(* Logix 5000 AddOnInstructionDefinition export; software revision 16.04 *)

TYPE AKD_Status :   // All connections to the drive ethernet module are established and data is successfully transferring.
STRUCT
   Profile_In_Progress : BOOL;   // Profile Move In Progress
   Block_In_Execution : BOOL;   // Block In Execution
   On_Target_Position : BOOL;   // On Target Position (1=Current Position Equals Last Target Position)
   General_Fault : BOOL;   // General Fault
   Current_Direction : BOOL;   // Current Motor Direction (0=Reverse, 1=Forward)
   Home_Level : BOOL;   // Level of Home Input
   Reg_Level : BOOL;   // Level of Registration Input
   Enable : BOOL;   // State of Enable Output
   Fault_Input_Fault : BOOL;   // Fault Input Active
   Fwd_Limit : BOOL;   // Forward Input Active
   Rev_Limit : BOOL;   // Reverse Input Active
   Positive_Limit : BOOL;   // Positive Software Limit Exceeded
   Negative_Limit : BOOL;   // Negative Software Limit Exceeded
   FE_Fault : BOOL;   // Following Error Fault
   Block_Fault : BOOL;   // Block Execution Fault
   Load_Complete : BOOL;   // Command Message Successfully Loaded
END_STRUCT
END_TYPE

TYPE AKD_Axis :   // Axis Data:
STRUCT
   Control : AKD_Control;   // Control bits to send to the drive
   Status : AKD_Status;   // Status bits received from the drive
   Input : AB:ETHERNET_MODULE_SINT_64Bytes:I:0;   // Data from the drive
   Output : AB:ETHERNET_MODULE_SINT_64Bytes:O:0;   // Data to the drive
   ResponseMsgType : SINT;   // Response type contained in latest IO response from drive. Used to check for errors
   CommandTimeout : INT;   // Time to allow for command response from drive. Dependent on scan rate and communicaiton rate
   PositionFeedback : DINT;   // Actual Position Value
   VelocityFeedback : DINT;   // Actual Velocity Value
END_STRUCT
END_TYPE

TYPE AKD_Control :   // Send Explicit Message
STRUCT
   Load_Data_Start_Profile : BOOL;   // Load Command Data / Start Profile Move
   Start_Block : BOOL;   // Execute Command block or block chain
   Incremental : BOOL;   // Incremental Position (0=Absolute, 1=Incremental)
   Direction : BOOL;   // Direction in Velocity Mode (0=Reverse, 1=Forward)
   Smooth_Stop : BOOL;   // Smooth / Controlled Stop w/ Deceleration
   Hard_Stop : BOOL;   // Hard / Immediate Stop
   Reg_Arm : BOOL;   // Arm the Registration Input
   Enable : BOOL;   // Enable Output
END_STRUCT
END_TYPE

ADD_ON_INSTRUCTION AKD_Disable   (* revision 2.1, ExecutePrescan, ExecuteEnableInFalse *)
// Disable Drive
// Revision note:
// Don't error if Command_Timeout preset is 0
VAR_OUTPUT
   DN : BOOL; {visible}   // Command Successful
   ER : BOOL; {visible}   // Error
END_VAR
VAR_IN_OUT
   Axis : AKD_Axis; {required}
END_VAR
VAR
   Command_Timeout : TIMER;   // Timeout Timer
END_VAR

ROUTINE EnableInFalse   (* ladder *)
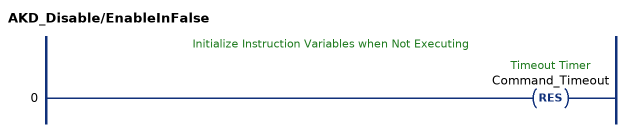
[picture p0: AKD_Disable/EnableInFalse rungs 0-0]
   // Initialize Instruction Variables when Not Executing
   0: RES(Command_Timeout);
END_ROUTINE

ROUTINE Logic   (* ladder *)
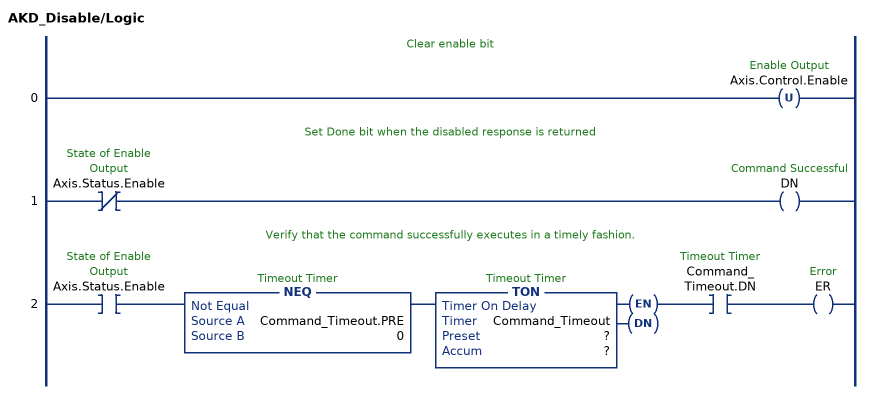
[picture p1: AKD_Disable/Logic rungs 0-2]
   // Clear enable bit
   0: OTU(Axis.Control.Enable);
   // Set Done bit when the disabled response is returned
   1: XIO(Axis.Status.Enable)OTE(DN);
   // Verify that the command successfully executes in a timely fashion.
   2: XIC(Axis.Status.Enable)NEQ(Command_Timeout.PRE,0)TON(Command_Timeout,?,?)XIC(Command_Timeout.DN)OTE(ER);
END_ROUTINE

ROUTINE Prescan   (* ladder *)
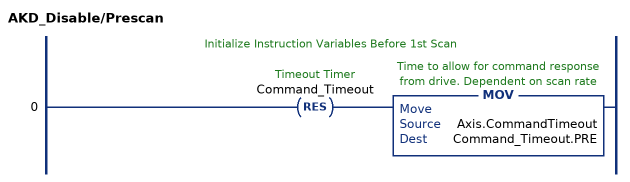
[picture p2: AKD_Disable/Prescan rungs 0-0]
   // Initialize Instruction Variables Before 1st Scan
   0: RES(Command_Timeout)MOV(Axis.CommandTimeout,Command_Timeout.PRE);
END_ROUTINE
END_ADD_ON_INSTRUCTION

ADD_ON_INSTRUCTION AKD_Set_Parameter   (* revision 2.0, ExecutePrescan, ExecuteEnableInFalse *)
// Set Drive Parameter
VAR_OUTPUT
   DN : BOOL; {visible}   // Command Successful
   ER : BOOL; {visible}   // Error
END_VAR
VAR_IN_OUT
   Axis : AKD_Axis; {required}
END_VAR
VAR_INPUT
   Parameter_Number : INT; {visible}   // See help (F1) for parameter list.
   Parameter_Value : DINT; {required}   // Parameter Value
END_VAR
VAR
   Command_Timeout : TIMER;   // Timeout Timer
   Command_Message_Type : SINT;   // Command Message Type
   Command_Axis_Number : SINT;   // Command Axis Number
   Step : SINT;
   Command_Bytes : SINT[8];
   OS_LoadStart : BOOL;
   Temp_Bytes : SINT[2];   // Temporary Bytes to Split into Command Bytes
END_VAR

ROUTINE EnableInFalse   (* ladder *)
// EnableIn_False
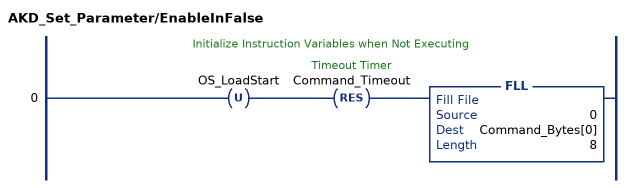
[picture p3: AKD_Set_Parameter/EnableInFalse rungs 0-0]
   // Initialize Instruction Variables when Not Executing
   0: OTU(OS_LoadStart)RES(Command_Timeout)FLL(0,Command_Bytes[0],8);
END_ROUTINE

ROUTINE Logic   (* ladder *)
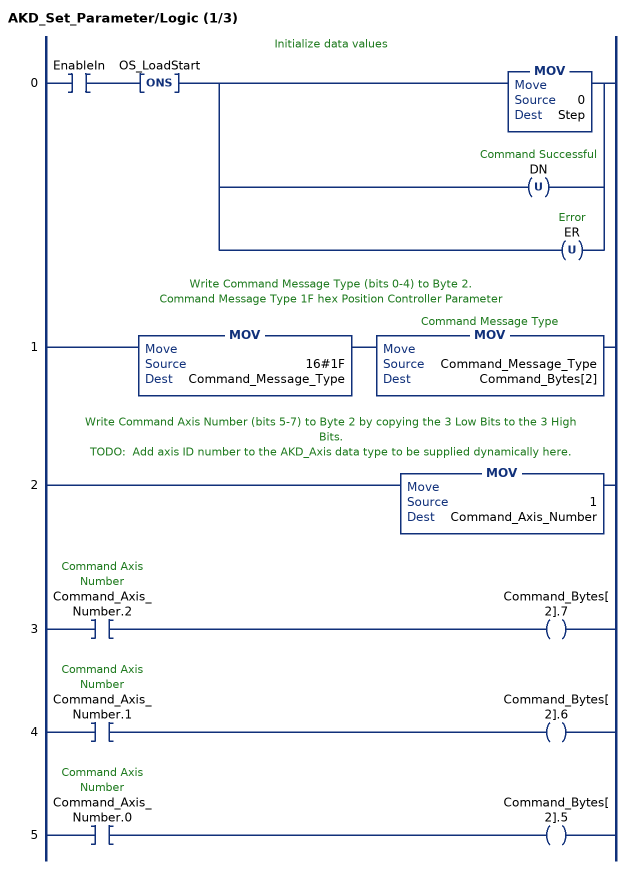
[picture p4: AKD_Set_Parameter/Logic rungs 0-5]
   // Initialize data values
   0: XIC(EnableIn)ONS(OS_LoadStart)[MOV(0,Step) ,OTU(DN) ,OTU(ER) ];
   // Write Command Message Type (bits 0-4) to Byte 2.
   // Command Message Type 1F hex Position Controller Parameter
   1: MOV(16#1F,Command_Message_Type)MOV(Command_Message_Type,Command_Bytes[2]);
   // Write Command Axis Number (bits 5-7) to Byte 2 by copying the 3 Low Bits to the 3 High Bits.
   // TODO:  Add axis ID number to the AKD_Axis data type to be supplied dynamically here.
   2: MOV(1,Command_Axis_Number);
   3: XIC(Command_Axis_Number.2)OTE(Command_Bytes[2].7);
   4: XIC(Command_Axis_Number.1)OTE(Command_Bytes[2].6);
   5: XIC(Command_Axis_Number.0)OTE(Command_Bytes[2].5);
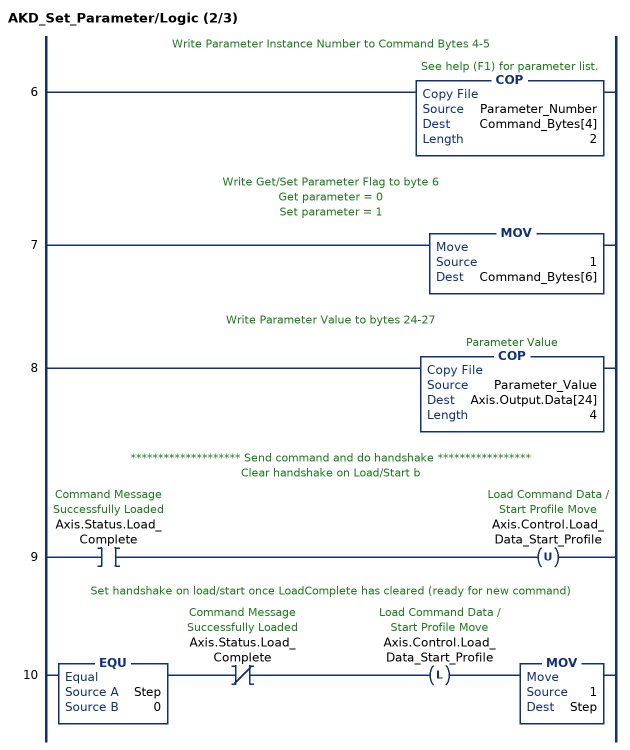
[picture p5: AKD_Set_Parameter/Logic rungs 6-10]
   // Write Parameter Instance Number to Command Bytes 4-5
   6: COP(Parameter_Number,Command_Bytes[4],2);
   // Write Get/Set Parameter Flag to byte 6
   // Get parameter = 0
   // Set parameter = 1
   7: MOV(1,Command_Bytes[6]);
   // Write Parameter Value to bytes 24-27
   8: COP(Parameter_Value,Axis.Output.Data[24],4);
   // ******************** Send command and do handshake *****************
   // Clear handshake on Load/Start b
   9: XIC(Axis.Status.Load_Complete)OTU(Axis.Control.Load_Data_Start_Profile);
   // Set handshake on load/start once LoadComplete has cleared (ready for new command)
   10: EQU(Step,0)XIO(Axis.Status.Load_Complete)OTL(Axis.Control.Load_Data_Start_Profile)MOV(1,Step);
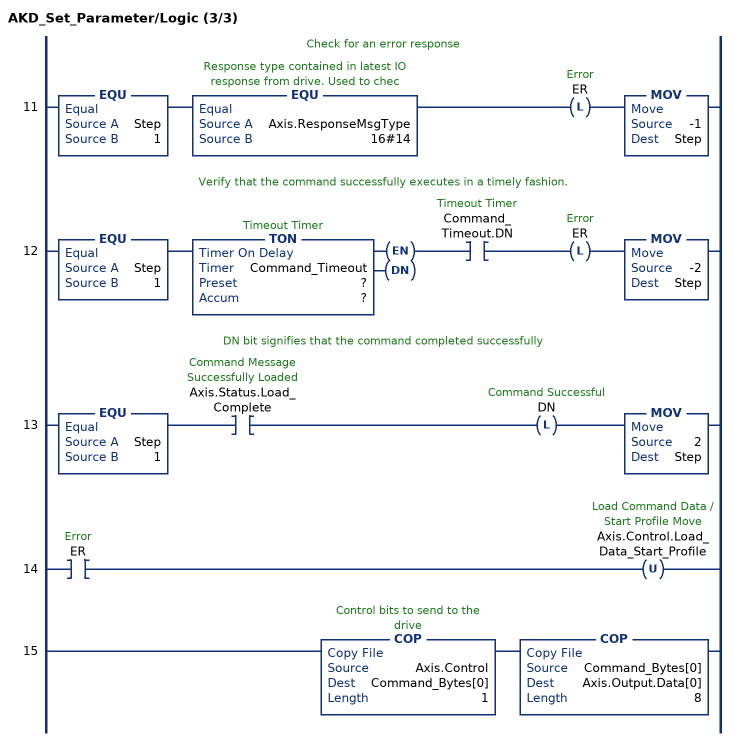
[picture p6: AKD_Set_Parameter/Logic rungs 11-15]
   // Check for an error response
   11: EQU(Step,1)EQU(Axis.ResponseMsgType,16#14)OTL(ER)MOV(-1,Step);
   // Verify that the command successfully executes in a timely fashion.
   12: EQU(Step,1)TON(Command_Timeout,?,?)XIC(Command_Timeout.DN)OTL(ER)MOV(-2,Step);
   // DN bit signifies that the command completed successfully
   13: EQU(Step,1)XIC(Axis.Status.Load_Complete)OTL(DN)MOV(2,Step);
   14: XIC(ER)OTU(Axis.Control.Load_Data_Start_Profile);
   15: COP(Axis.Control,Command_Bytes[0],1)COP(Command_Bytes[0],Axis.Output.Data[0],8);
END_ROUTINE

ROUTINE Prescan   (* ladder *)
// Prescan
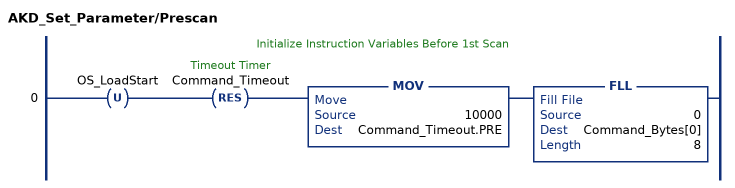
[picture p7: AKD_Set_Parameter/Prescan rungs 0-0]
   // Initialize Instruction Variables Before 1st Scan
   0: OTU(OS_LoadStart)RES(Command_Timeout)MOV(10000,Command_Timeout.PRE)FLL(0,Command_Bytes[0],8);
END_ROUTINE
END_ADD_ON_INSTRUCTION

ADD_ON_INSTRUCTION AKD_Fault_Reset   (* revision 2.0, ExecutePrescan, ExecuteEnableInFalse *)
// Drive Fault Reset
VAR_OUTPUT
   DN : BOOL; {visible}   // Command Successful
   ER : BOOL; {visible}   // Error
END_VAR
VAR_IN_OUT
   Axis : AKD_Axis; {required}
END_VAR
VAR
   Step : SINT;
   Set_Parameter : AKD_Set_Parameter;
END_VAR

ROUTINE EnableInFalse   (* ladder *)
// EnableIn_False
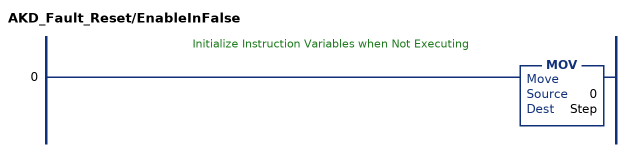
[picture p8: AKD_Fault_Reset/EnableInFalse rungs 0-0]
   // Initialize Instruction Variables when Not Executing
   0: MOV(0,Step);
END_ROUTINE

ROUTINE Logic   (* ladder *)
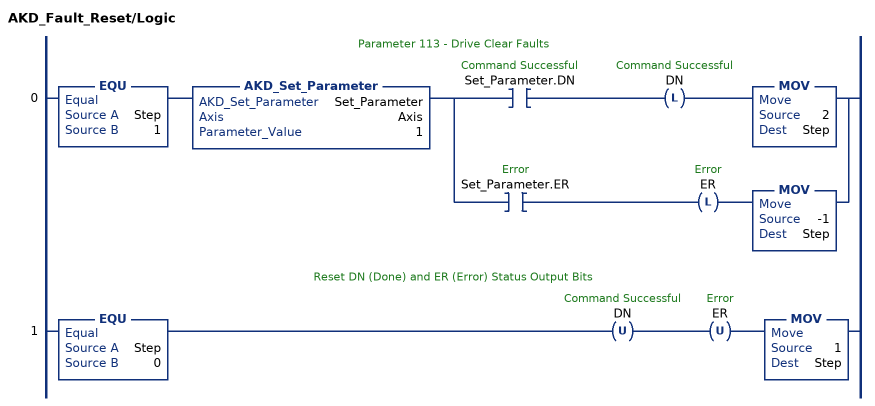
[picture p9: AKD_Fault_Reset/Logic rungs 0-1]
   // Parameter 113 - Drive Clear Faults
   0: EQU(Step,1)AKD_Set_Parameter(Set_Parameter,Axis,1)[XIC(Set_Parameter.DN) OTL(DN) MOV(2,Step) ,XIC(Set_Parameter.ER) OTL(ER) MOV(-1,Step) ];
   // Reset DN (Done) and ER (Error) Status Output Bits
   1: EQU(Step,0)OTU(DN)OTU(ER)MOV(1,Step);
END_ROUTINE

ROUTINE Prescan   (* ladder *)
// Prescan
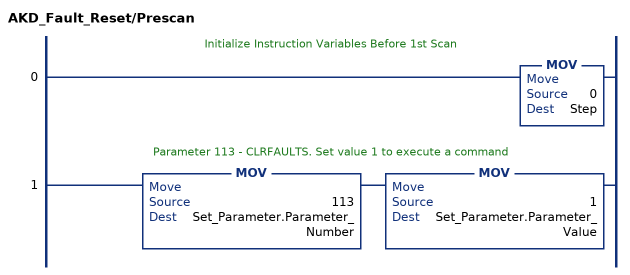
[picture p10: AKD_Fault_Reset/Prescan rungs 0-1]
   // Initialize Instruction Variables Before 1st Scan
   0: MOV(0,Step);
   // Parameter 113 - CLRFAULTS. Set value 1 to execute a command
   1: MOV(113,Set_Parameter.Parameter_Number)MOV(1,Set_Parameter.Parameter_Value);
END_ROUTINE
END_ADD_ON_INSTRUCTION

ADD_ON_INSTRUCTION AKD_Shutdown_Reset   (* revision 2.1, ExecutePrescan, ExecuteEnableInFalse *)
// Reset Drive after a Shutdown Command
// Revision note:
// Set disable timeout to 100ms
VAR_OUTPUT
   DN : BOOL; {visible}   // Command Successful
   ER : BOOL; {visible}   // Error
END_VAR
VAR_IN_OUT
   Axis : AKD_Axis; {required}
END_VAR
VAR
   Fault_Reset : AKD_Fault_Reset;
   Set_Disable : AKD_Disable;
   Step : SINT;   // Sequence Step Number
   OS_Start_Sequence : BOOL;
   Command_Timeout : TIMER;
   Disable_Timer : TIMER;
END_VAR

ROUTINE EnableInFalse   (* ladder *)
// EnableIn_False
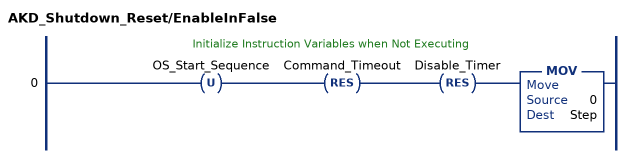
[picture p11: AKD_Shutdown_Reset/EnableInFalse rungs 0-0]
   // Initialize Instruction Variables when Not Executing
   0: OTU(OS_Start_Sequence)RES(Command_Timeout)RES(Disable_Timer)MOV(0,Step);
END_ROUTINE

ROUTINE Logic   (* ladder *)
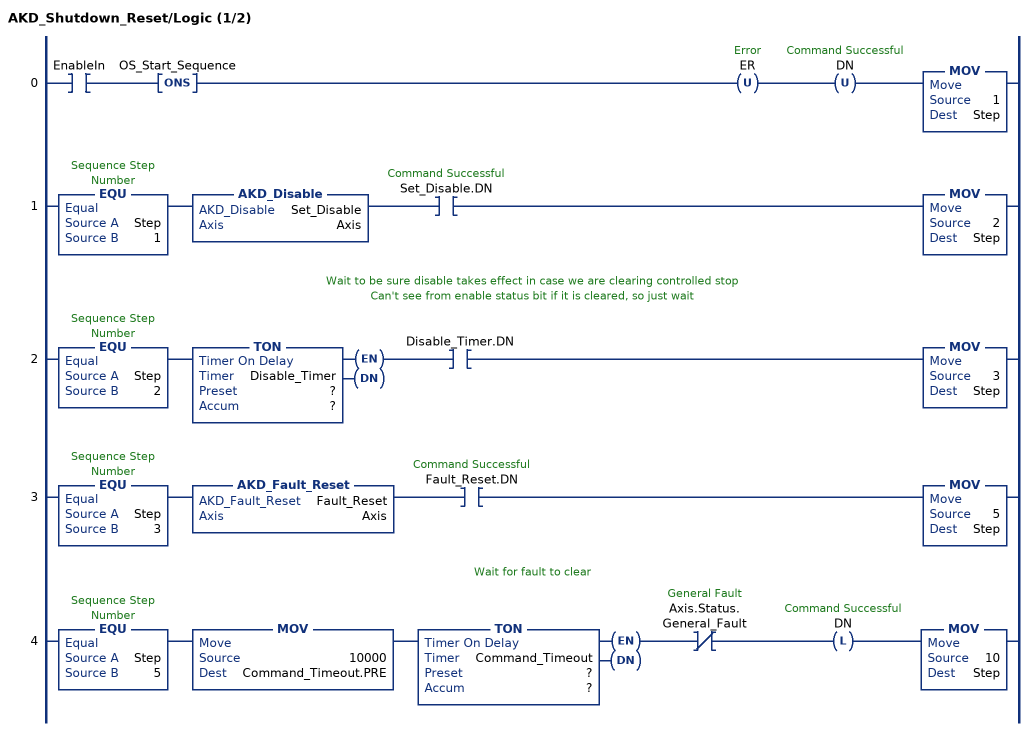
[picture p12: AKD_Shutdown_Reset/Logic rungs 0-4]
   0: XIC(EnableIn)ONS(OS_Start_Sequence)OTU(ER)OTU(DN)MOV(1,Step);
   1: EQU(Step,1)AKD_Disable(Set_Disable,Axis)XIC(Set_Disable.DN)MOV(2,Step);
   // Wait to be sure disable takes effect in case we are clearing controlled stop
   // Can't see from enable status bit if it is cleared, so just wait
   2: EQU(Step,2)TON(Disable_Timer,?,?)XIC(Disable_Timer.DN)MOV(3,Step);
   3: EQU(Step,3)AKD_Fault_Reset(Fault_Reset,Axis)XIC(Fault_Reset.DN)MOV(5,Step);
   // Wait for fault to clear
   4: EQU(Step,5)MOV(10000,Command_Timeout.PRE)TON(Command_Timeout,?,?)XIO(Axis.Status.General_Fault)OTL(DN)MOV(10,Step);
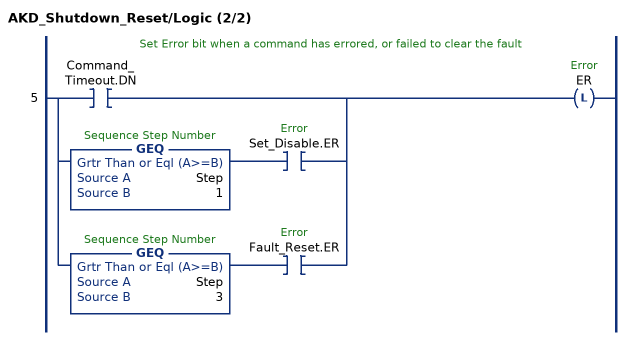
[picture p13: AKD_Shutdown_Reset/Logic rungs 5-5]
   // Set Error bit when a command has errored, or failed to clear the fault
   5: [XIC(Command_Timeout.DN) ,GEQ(Step,1) XIC(Set_Disable.ER) ,GEQ(Step,3) XIC(Fault_Reset.ER) ]OTL(ER);
END_ROUTINE

ROUTINE Prescan   (* ladder *)
// Prescan
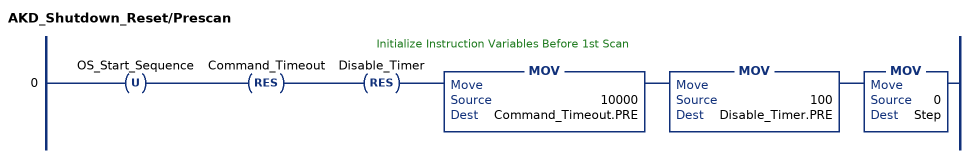
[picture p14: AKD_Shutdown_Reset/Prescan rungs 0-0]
   // Initialize Instruction Variables Before 1st Scan
   0: OTU(OS_Start_Sequence)RES(Command_Timeout)RES(Disable_Timer)MOV(10000,Command_Timeout.PRE)MOV(100,Disable_Timer.PRE)MOV(0,Step);
END_ROUTINE
END_ADD_ON_INSTRUCTION
